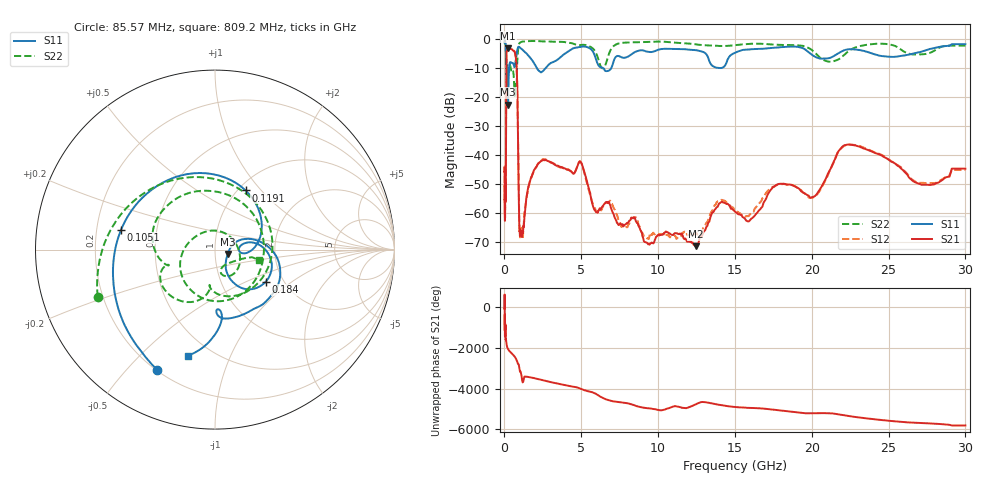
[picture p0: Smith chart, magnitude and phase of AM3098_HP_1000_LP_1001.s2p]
! Date/Time: Thu, Feb 28, 2019 8:40 AM
! Network Analyzer: Agilent Technologies E8364B Rev: A.07.50.67
! Sweep from 0.010 to 30.000 GHz, 1601 Points, Sweep Type: LOG
! Power Supply: 5.023 V, 0.002 A
# Hz S DB R 50
!freq MagS11 AngS11 MagS21 AngS21 MagS12 AngS12 MagS22 AngS22
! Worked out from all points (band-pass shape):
!   1601 points, 10 MHz to 30 GHz, reference 50 ohm
!   highest |S21| = -3.04 dB at 241.1 MHz (marker M1); lowest = -71.4 dB at 12.43 GHz (marker M2)
!   |S21| within 3 dB of the highest: 128 MHz to 735.1 MHz (607.2 MHz wide, 141 % of centre)
!   lowest |S11| = -22.5 dB at 238.7 MHz (marker M3), VSWR 1.16, Z = 57.6 - j2.82 ohm
!   |S11| at or under -10 dB: 191.3 MHz to 302.1 MHz (110.8 MHz wide, 44.9 % of centre); 2.119 GHz to 2.666 GHz (547.3 MHz wide, 22.9 % of centre); 6.456 GHz to 6.939 GHz (482.9 MHz wide, 7.21 % of centre)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
!   |S22| runs from -19.8 to -0.5 dB; largest |S21 - S12| = 0.011
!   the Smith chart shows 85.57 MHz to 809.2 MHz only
!   S11 on the Smith chart (normalised r, x): 85.57 MHz: 0.20, -0.61; 105.1 MHz: 0.31, +0.09; 119.1 MHz: 1.08, +0.83; 184 MHz: 1.62, -0.65; 809.2 MHz: 0.37, -0.71
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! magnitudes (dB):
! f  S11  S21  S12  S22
! 10 MHz  -0.4  -45.8  -44.3  -0.6
! 38.04 MHz  -0.5  -60.7  -57.7  -0.9
! 49.1 MHz  -0.8  -52.4  -47.4  -1.3
! 85.57 MHz  -2.6  -54.2  -52.3  -3.0
! 105.1 MHz  -5.4  -27.1  -27.1  -7.0
! 119.1 MHz  -8.6  -10.3  -10.3  -10.2
! 144.7 MHz  -16.8  -4.2  -4.2  -13.1
! 184 MHz  -9.5  -3.6  -3.6  -8.9
! 238.7 MHz  -22.5  -3.0  -3.0  -11.3
! 241.1 MHz  -22.4  -3.0  -3.0  -11.3
! 317.5 MHz  -9.0  -3.3  -3.2  -8.9
! 550.5 MHz  -8.2  -3.8  -3.8  -10.8
! 809.2 MHz  -4.3  -11.8  -11.8  -11.9
! 949.8 MHz  -2.6  -61.4  -58.9  -1.5
! 1.019 GHz  -2.9  -67.8  -68.3  -1.1
! 2.084 GHz  -9.6  -44.0  -43.9  -0.6
! 4.927 GHz  -2.5  -42.1  -42.1  -1.9
! 7.926 GHz  -6.2  -63.7  -64.7  -1.1
! 12.43 GHz  -3.7  -71.4  -67.0  -1.7
! 20.1 GHz  -5.6  -54.3  -54.5  -4.1
! 22.56 GHz  -3.4  -36.4  -36.3  -3.5
! 30 GHz  -1.6  -44.6  -45.0  -2.1
